FUNCTION "DIVE" : VOID
TITLE =
VERSION : 0.1


VAR_TEMP
  zero : BOOL ;
END_VAR
BEGIN
NETWORK
TITLE =Produzione in corso
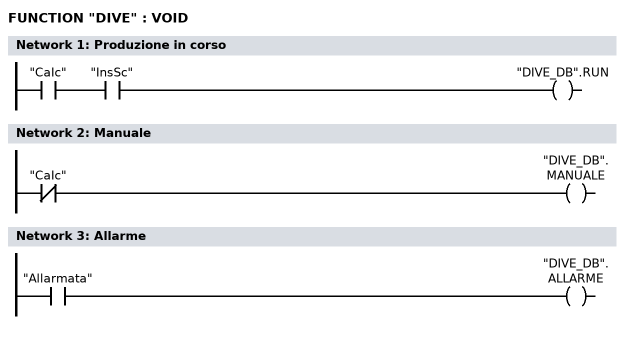
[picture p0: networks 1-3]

      U     "CaIc";
      U     "InsSc";
      =     "DIVE_DB".RUN;
NETWORK
TITLE =Manuale

      UN    "CaIc";
      =     "DIVE_DB".MANUALE;
NETWORK
TITLE =Allarme

      U     "Allarmata";
      =     "DIVE_DB".ALLARME;
NETWORK
TITLE =Bit sempre a zero


      CLR   ;
      =     "ALWAYS_0";
      U     "ALWAYS_0";
      =     #zero;
NETWORK
TITLE =Mancato Carico
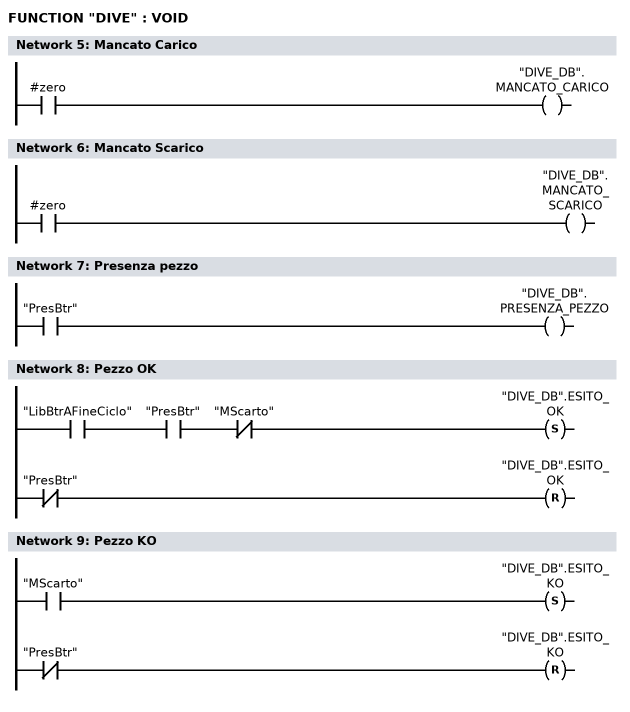
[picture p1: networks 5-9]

      U     #zero;
      =     "DIVE_DB".MANCATO_CARICO;
NETWORK
TITLE =Mancato Scarico

      U     #zero;
      =     "DIVE_DB".MANCATO_SCARICO;
NETWORK
TITLE =Presenza pezzo

      U     "PresBtr";
      =     "DIVE_DB".PRESENZA_PEZZO;
NETWORK
TITLE =Pezzo OK

      U     "LibBtrAFineCiclo";
      U     "PresBtr";
      UN    "MScarto";
      S     "DIVE_DB".ESITO_OK;
      UN    "PresBtr";
      R     "DIVE_DB".ESITO_OK;
      NOP   0;
NETWORK
TITLE =Pezzo KO

      U     "MScarto";
      S     "DIVE_DB".ESITO_KO;
      UN    "PresBtr";
      R     "DIVE_DB".ESITO_KO;
      NOP   0;
NETWORK
TITLE =Fine Lavoro

      U(    ;
      U(    ;
      O     "LibBtrAFineCiclo";
      O     "MScarto";
      )     ;
      S     "M6.3";
      UN    "PresBtr";
      R     "M6.3";
      U     "M6.3";
      )     ;
      L     S5T#500MS;
      SE    T     25;
      NOP   0;
      NOP   0;
      NOP   0;
      U     T     25;
      =     "DIVE_DB".FINE_LAVORO;
NETWORK
TITLE =Inizio Pallet
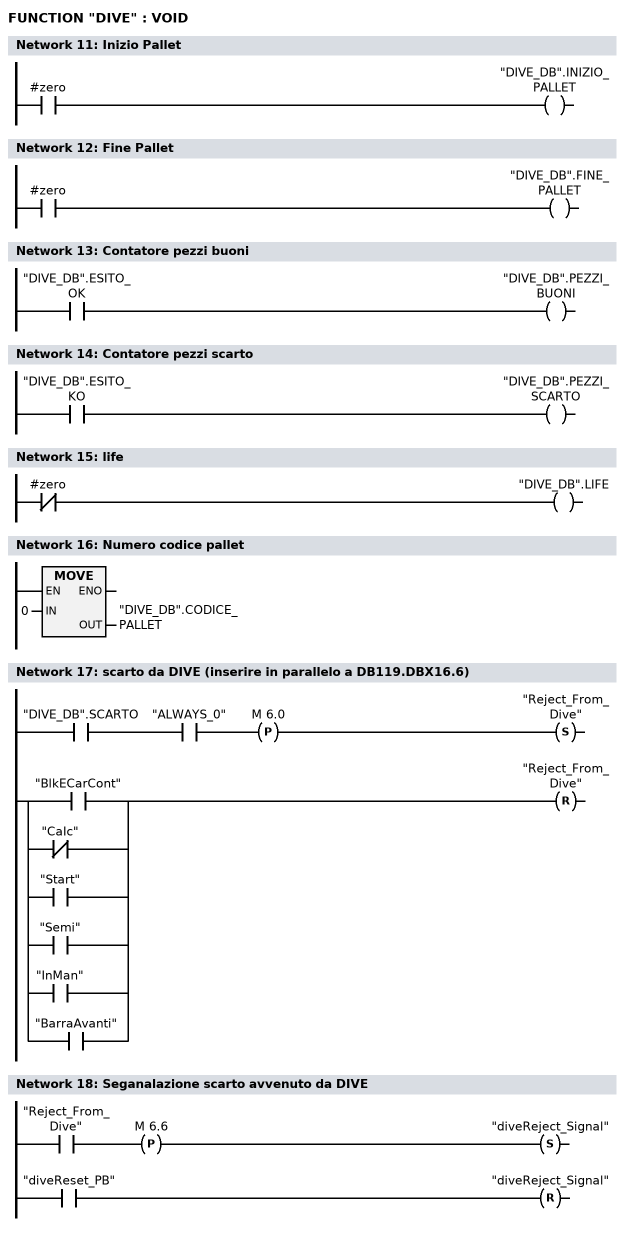
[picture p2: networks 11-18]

      U     #zero;
      =     "DIVE_DB".INIZIO_PALLET;
NETWORK
TITLE =Fine Pallet

      U     #zero;
      =     "DIVE_DB".FINE_PALLET;
NETWORK
TITLE =Contatore pezzi buoni

      U     "DIVE_DB".ESITO_OK;
      =     "DIVE_DB".PEZZI_BUONI;
NETWORK
TITLE =Contatore pezzi scarto

      U     "DIVE_DB".ESITO_KO;
      =     "DIVE_DB".PEZZI_SCARTO;
NETWORK
TITLE =life

      UN    #zero;
      =     "DIVE_DB".LIFE;
NETWORK
TITLE =Numero codice pallet

      L     0;
      T     "DIVE_DB".CODICE_PALLET;
      NOP   0;
NETWORK
TITLE =scarto da DIVE (inserire in parallelo a DB119.DBX16.6)

      U     "DIVE_DB".SCARTO;
      U     "ALWAYS_0";
      FP    M      6.0;
      S     "Reject_From_Dive";
      U(    ;
      O     "BlkECarCont";
      ON    "CaIc";
      O     "Start";
      O     "Semi";
      O     "InMan";
      O     "BarraAvanti";
      )     ;
      R     "Reject_From_Dive";
      NOP   0;
NETWORK
TITLE =Seganalazione scarto avvenuto da DIVE

      U     "Reject_From_Dive";
      FP    M      6.6;
      S     "diveReject_Signal";
      U     "diveReset_PB";
      R     "diveReject_Signal";
      NOP   0;
END_FUNCTION

